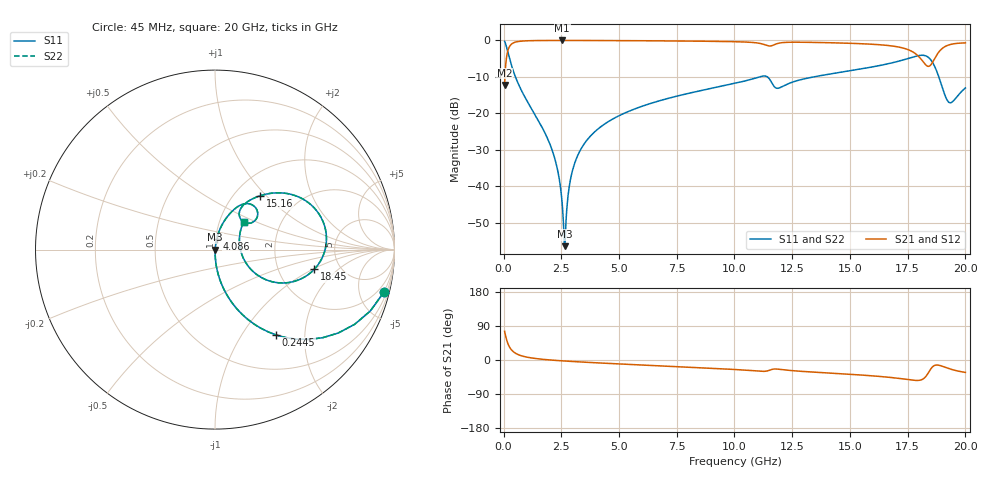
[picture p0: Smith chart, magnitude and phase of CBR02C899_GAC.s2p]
! S-parameter model data by Modelithics Inc.  support@modelithics.com 813-866-6335  Tampa FL USA
! S-Parameter data specifications:
! Substrate: 20-mil Rogers 4350B, substrate thickness, H=0.508mm, Dielectric constant, Er=3.75
! PCB Mounting Pad Footprint: Pad width, PadW=0.32mm , Pad length, PadL=0.37mm , Pad gap, PadG (edge-to-edge)=0.19mm , Reference planes=0.93mm apart
#  GHz  S  MA  R 50
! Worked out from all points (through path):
!   801 points, 45 MHz to 20 GHz, reference 50 ohm
!   highest |S21| = -0.01 dB at 2.539 GHz (marker M1); lowest = -12.2 dB at 45 MHz (marker M2)
!   group delay of S21, straight-line fit = 7.32 ps
!   lowest |S11| = -56.5 dB at 2.639 GHz (marker M3), VSWR 1.00, Z = 50.1 - j0.0409 ohm
!   |S11| at or under -10 dB: 513.6 MHz to 11.08 GHz (10.56 GHz wide, 182 % of centre); 11.42 GHz to 13.44 GHz (2.017 GHz wide, 16.2 % of centre); 18.85 GHz to end of sweep
!   |S22| runs from -56.5 to -0.3 dB; largest |S21 - S12| = 0
!   S11 on the Smith chart (normalised r, x): 45 MHz: 0.99, -7.88; 244.6 MHz: 1.00, -1.44; 4.086 GHz: 1.01, +0.12; 15.16 GHz: 1.30, +0.92; 18.45 GHz: 3.22, -1.04; 20 GHz: 1.30, +0.42
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0.045  0.9694 -14.2  0.2452 75.8  0.2452 75.8  0.9694 -14.2
0.24455  0.5849 -54.4  0.8106 35.5  0.8106 35.5  0.5849 -54.4
0.668594  0.2417 -76.5  0.9695 13.3  0.9695 13.3  0.2417 -76.5
2.090387  0.03207 -87.9  0.9981 -0.3  0.9981 -0.3  0.03207 -87.9
2.389712  0.01383 -85.8  0.9985 -1.6  0.9985 -1.6  0.01383 -85.8
2.539375  0.005727 -77.7  0.9985 -2.3  0.9985 -2.3  0.005727 -77.7
2.63915  0.001503 -15.8  0.9985 -2.7  0.9985 -2.7  0.001503 -15.8
2.963419  0.01543 80.4  0.9983 -3.9  0.9983 -3.9  0.01543 80.4
3.387462  0.03382 81.9  0.9977 -5.4  0.9977 -5.4  0.03382 81.9
4.085888  0.06085 80.7  0.9963 -7.6  0.9963 -7.6  0.06085 80.7
6.704981  0.1471 73.8  0.9867 -15.2  0.9867 -15.2  0.1471 73.8
10.0225  0.2578 63.5  0.9598 -25.1  0.9598 -25.1  0.2578 63.5
11.29463  0.3256 47.3  0.8761 -29.9  0.8761 -29.9  0.3256 47.3
11.89328  0.2208 48.6  0.9119 -24.2  0.9119 -24.2  0.2208 48.6
13.36496  0.3129 56.4  0.9397 -31.7  0.9397 -31.7  0.3129 56.4
15.16091  0.3908 50.1  0.9096 -38.3  0.9096 -38.3  0.3908 50.1
16.68248  0.4807 41.1  0.8495 -45.6  0.8495 -45.6  0.4807 41.1
17.75506  0.5945 24.1  0.6856 -53.5  0.6856 -53.5  0.5945 24.1
18.45349  0.5637 -11.3  0.4466 -28.1  0.4466 -28.1  0.5637 -11.3
18.75281  0.3814 -28.6  0.6268 -13.2  0.6268 -13.2  0.3814 -28.6
19.27663  0.1422 -1.1  0.8658 -22.5  0.8658 -22.5  0.1422 -1.1
20  0.2226 43.9  0.9247 -32.8  0.9247 -32.8  0.2226 43.9
